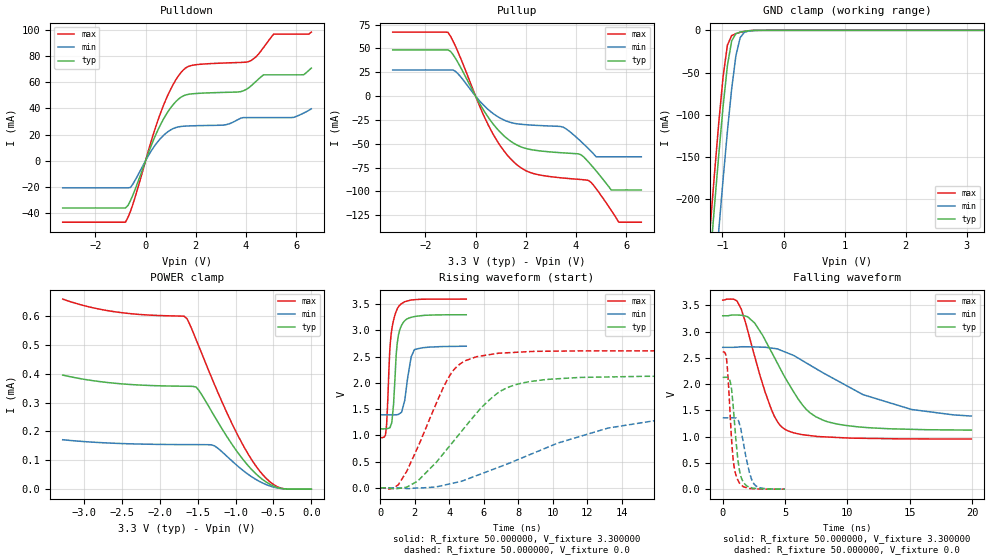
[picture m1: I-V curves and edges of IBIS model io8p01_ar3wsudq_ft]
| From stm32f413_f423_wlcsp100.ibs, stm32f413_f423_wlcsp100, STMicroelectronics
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|   Model io8p01_ar3wsudq_ft
[Model]  io8p01_ar3wsudq_ft
Model_type I/O
Polarity   Non-Inverting
Enable   Active-Low
Vinl =   0.990000V
Vinh =   2.310000V
Vmeas =  1.650000V
Cref =   50.000000pF
Rref =   100.000000M
Vref =   0.0V
C_comp   3.843200pF   3.762100pF   3.937000pF
[Temperature Range]   25.000000   0.125000k   -40.000000
[Pullup Reference]   3.300000V   2.700000V   3.600000V
[Pulldown Reference]   0.0V   0.0V   0.0V
[POWER Clamp Reference]   3.300000V   2.700000V   3.600000V
[GND Clamp Reference]   0.0V   0.0V   0.0V
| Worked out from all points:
|   slope of the pulldown table from 0 to 0.495 V, typ, clamps not added: 20.9 ohm
|   slope of the pullup table from 0 to 0.495 V, typ, clamps not added: 22.6 ohm
|   GND clamp passes 1 mA (typ) near -0.62 V on its own axis
|   rising waveform, R_fixture 50.000000, V_fixture 3.300000: 20-80 % time 270ps typ, 352ps min, 283ps max; typ from 1.12 V to 3.3 V
|   rising waveform, R_fixture 50.000000, V_fixture 0.0: 20-80 % time 3.35ns typ, 6.78ns min, 2.11ns max; typ from 0 V to 2.13 V
|   falling waveform, R_fixture 50.000000, V_fixture 3.300000: 20-80 % time 3.21ns typ, 6.81ns min, 2.02ns max; typ from 3.3 V to 1.12 V
|   falling waveform, R_fixture 50.000000, V_fixture 0.0: 20-80 % time 505ps typ, 698ps min, 426ps max; typ from 2.13 V to 0 V
[Pulldown]
|Voltage   I(typ)   I(min)   I(max)
-3.3V     -36.18mA   -20.77mA   -47.07mA
-800mV    -36.18mA   -20.77mA   -47.07mA
-600mV    -30.5mA    -20.52mA   -38.69mA
700mV     31.4mA     19.11mA    41.71mA
1.2V      45.15mA    25.37mA    61.75mA
1.6V      50.35mA    26.5mA     71.06mA
3.1V      52.28mA    27.26mA    74.76mA
4.1V      55.71mA    33.01mA    75.8mA
4.7V      65.73mA    33.01mA    86.69mA
5.1V      65.73mA    33.01mA    96.9mA
6.3V      65.85mA    36.5mA     96.9mA
6.6V      70.91mA    39.71mA    98.45mA
[Pullup]
|Voltage   I(typ)   I(min)   I(max)
-3.3V     48.54mA    27.45mA    67.16mA
-1.1V     48.54mA    27.45mA    66.88mA
-700mV    35.13mA    23.48mA    46.33mA
500mV     -22.07mA   -14mA      -30.03mA
1.5V      -49.1mA    -28.3mA    -68.56mA
2.2V      -56.05mA   -30.32mA   -80.35mA
3.5V      -59.53mA   -32.72mA   -85.92mA
4.5V      -69.21mA   -55.27mA   -88.43mA
4.8V      -78.37mA   -63.6mA    -97.01mA
5.4V      -98.4mA    -63.6mA    -119.7mA
5.7V      -98.4mA    -63.6mA    -132.2mA
6.6V      -98.4mA    -63.6mA    -132.2mA
[GND_clamp]
|Voltage   I(typ)   I(min)   I(max)
-3.3V     -2.327A    -2.405A    -2.301A
-1.2V     -270.2mA   -361.4mA   -232.1mA
-1.13V    -207.3mA   -298.1mA   -169mA
-1.06V    -146.7mA   -236.2mA   -108.8mA
-990mV    -90.18mA   -176.4mA   -54.96mA
-920mV    -42.21mA   -120mA     -17.68mA
-850mV    -12.57mA   -69.47mA   -6.265mA
-780mV    -3.971mA   -30.01mA   -3.886mA
-710mV    -2.1mA     -8.615mA   -2.382mA
-640mV    -1.148mA   -2.283mA   -1.22mA
-570mV    -524uA     -821.5uA   -476.8uA
3.28V     0A         0A         0A
[POWER_clamp]
|Voltage   I(typ)   I(min)   I(max)
-3.28V    395.3uA    171.3uA    658.7uA
-2.6V     367.1uA    159uA      614.9uA
-1.68V    356.7uA    154.4uA    599.4uA
-1.64V    356.5uA    154.4uA    590.8uA
-1.52V    353.6uA    154.3uA    518.3uA
-1.48V    341.1uA    154.2uA    492.3uA
-1.28V    253.6uA    150.4uA    364.2uA
-960mV    123.1uA    77.56uA    181.6uA
-720mV    50.52uA    32.03uA    76.18uA
-560mV    18.94uA    12.27uA    28.65uA
-440mV    5.104uA    3.69uA     7.327uA
0V        0A         0A         0A
[Ramp]
| variable   typ   min   max
dV/dt_r  1.27866/3.35822n   0.79836/6.76710n   1.56750/2.11322n
dV/dt_f  1.30236/3.21183n   0.74070/6.78201n   1.58789/2.02042n
R_load = 50.000000
[Rising Waveform]
R_fixture= 50.000000
V_fixture= 3.300000
V_fixture_min= 2.700000
V_fixture_max= 3.600000
|time   V(typ)   V(min)   V(max)
0s        1.124V     1.392V     954.3mV
360.4ps   1.127V     1.392V     1.185V
550.6ps   1.144V     1.392V     2.616V
660.7ps   1.236V     1.392V     3.001V
930.9ps   2.57V      1.393V     3.371V
1.031ns   2.864V     1.397V     3.44V
1.411ns   3.183V     1.657V     3.548V
1.782ns   3.25V      2.479V     3.581V
1.982ns   3.265V     2.636V     3.587V
4.985ns   3.3V       2.7V       3.599V
[Rising Waveform]
R_fixture= 50.000000
V_fixture= 0.0
V_fixture_min= 0.0
V_fixture_max= 0.0
|time   V(typ)   V(min)   V(max)
0s        357.1uV    204.2uV    681.8uV
1.041ns   -12.84mV   -1.324mV   56.46mV
2.162ns   126.4mV    -3.368mV   765.8mV
3.844ns   725.9mV    60.55mV    2.034V
4.364ns   935.7mV    98.86mV    2.286V
5.005ns   1.196V     160.8mV    2.433V
6.807ns   1.808V     384.8mV    2.564V
8.649ns   2.025V     629.1mV    2.597V
13.21ns   2.114V     1.139V     2.611V
19.94ns   2.129V     1.359V     2.612V
[Falling Waveform]
R_fixture= 50.000000
V_fixture= 3.300000
V_fixture_min= 2.700000
V_fixture_max= 3.600000
|time   V(typ)   V(min)   V(max)
0s        3.3V       2.7V       3.599V
920.9ps   3.315V     2.7V       3.612V
1.481ns   3.31V      2.71V      3.431V
2.563ns   3.162V     2.707V     2.529V
3.804ns   2.66V      2.689V     1.581V
5.045ns   2.107V     2.607V     1.133V
6.687ns   1.522V     2.405V     1.029V
8.368ns   1.286V     2.173V     993.3mV
15.14ns   1.139V     1.518V     956.6mV
19.94ns   1.124V     1.392V     954.3mV
[Falling Waveform]
R_fixture= 50.000000
V_fixture= 0.0
V_fixture_min= 0.0
V_fixture_max= 0.0
|time   V(typ)   V(min)   V(max)
0s        2.129V     1.359V     2.612V
300.3ps   2.13V      1.359V     2.49V
470.5ps   2.118V     1.358V     1.966V
620.6ps   2.031V     1.358V     1.318V
840.8ps   1.577V     1.36V      560.5mV
1.201ns   598.8mV    1.32V      179.6mV
1.592ns   161.9mV    968.2mV    58.09mV
2.152ns   36.98mV    305.7mV    13.54mV
2.472ns   18.5mV     112.7mV    8.776mV
4.985ns   357.1uV    204.2uV    681.8uV
